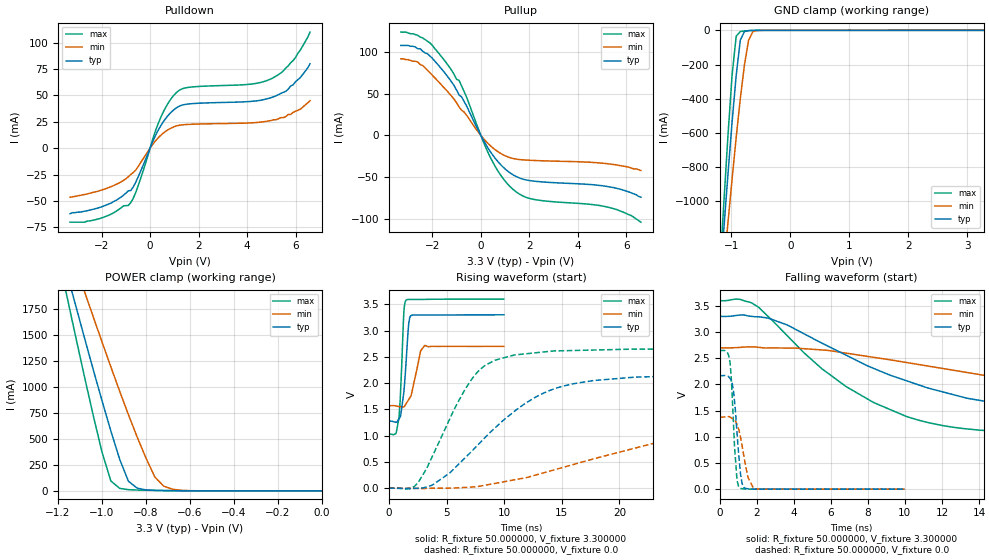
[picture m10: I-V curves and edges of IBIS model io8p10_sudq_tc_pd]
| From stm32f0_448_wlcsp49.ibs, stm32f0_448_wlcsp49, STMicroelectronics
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|   Model io8p10_sudq_tc_pd
[Model]  io8p10_sudq_tc_pd
Model_type I/O
Polarity   Non-Inverting
Enable   Active-Low
Vinl =   0.990000V
Vinh =   2.310000V
Vmeas =  1.650000V
Cref =   50.000000pF
Rref =   100.000000M
Vref =   0.0V
C_comp   1.329900pF   1.255600pF   1.431200pF
[Temperature Range]   25.000000   0.125000k   -40.000000
[Pullup Reference]   3.300000V   2.700000V   3.600000V
[Pulldown Reference]   0.0V   0.0V   0.0V
[POWER Clamp Reference]   3.300000V   2.700000V   3.600000V
[GND Clamp Reference]   0.0V   0.0V   0.0V
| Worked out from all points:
|   slope of the pulldown table from 0 to 0.495 V, typ, clamps not added: 21.3 ohm
|   slope of the pullup table from 0 to 0.495 V, typ, clamps not added: 20.9 ohm
|   GND clamp passes 1 mA (typ) near -0.66 V on its own axis
|   POWER clamp passes 1 mA (typ) near -0.60 V on its own axis
|   rising waveform, R_fixture 50.000000, V_fixture 3.300000: 20-80 % time 430ps typ, 663ps min, 305ps max; typ from 1.27 V to 3.3 V
|   rising waveform, R_fixture 50.000000, V_fixture 0.0: 20-80 % time 6.79ns typ, 16.1ns min, 3.73ns max; typ from 0 V to 2.17 V
|   falling waveform, R_fixture 50.000000, V_fixture 3.300000: 20-80 % time 9.37ns typ, 15.7ns min, 5.83ns max; typ from 3.3 V to 1.27 V
|   falling waveform, R_fixture 50.000000, V_fixture 0.0: 20-80 % time 301ps typ, 442ps min, 235ps max; typ from 2.17 V to 0 V
[Pulldown]
|Voltage   I(typ)   I(min)   I(max)
-3.3V     -62mA      -46.4mA    -70mA
-2.1V     -56.2mA    -40.3mA    -66.8mA
-800mV    -40.04mA   -24.9mA    -51.58mA
-500mV    -27.57mA   -17.6mA    -36.07mA
400mV     19.71mA    11.36mA    27.01mA
700mV     29.83mA    16.93mA    40.97mA
1.1V      38.46mA    21.2mA     53.02mA
1.6V      41.98mA    22.62mA    57.7mA
4.1V      44.26mA    24mA       60.59mA
5V        48mA       26.3mA     65.8mA
5.9V      60mA       34mA       83mA
6.6V      80mA       45mA       110mA
[Pullup]
|Voltage   I(typ)   I(min)   I(max)
-3.3V     108mA      92mA       124mA
-2.6V     104mA      88mA       120mA
-2.2V     98mA       78.2mA     113mA
-1.4V     71.8mA     53.6mA     86.1mA
-900mV    48.51mA    34.23mA    66.14mA
-700mV    41.33mA    28.36mA    53.31mA
400mV     -19.77mA   -12.52mA   -26.8mA
900mV     -37.48mA   -22.89mA   -50.99mA
1.4V      -48.39mA   -28.06mA   -66.43mA
2.2V      -54.79mA   -29.98mA   -76.75mA
5.3V      -61.7mA    -34.2mA    -86.4mA
6.6V      -74mA      -42mA      -104mA
[GND_clamp]
|Voltage   I(typ)   I(min)   I(max)
-3.3V     -9.739A    -9.975A    -9.587A
-1.2V     -1.489A    -1.65A     -1.416A
-1.13V    -1.162A    -1.385A    -1.009A
-1.06V    -842.3mA   -1.125A    -616.9mA
-990mV    -537.1mA   -870.2mA   -263mA
-920mV    -262.5mA   -625.3mA   -33.98mA
-850mV    -56.96mA   -397.5mA   -7.097mA
-780mV    -7.026mA   -202.3mA   -3.727mA
-710mV    -1.792mA   -58.24mA   -1.753mA
-640mV    -564.1uA   -8.795mA   -558.4uA
-570mV    -123.3uA   -1.303mA   -102.2uA
3.28V     84.11uA    64.12uA    93.81uA
[POWER_clamp]
|Voltage   I(typ)   I(min)   I(max)
-3.28V    9.897A     9.838A     9.594A
-1.16V    2.103A     2.419A     1.88A
-1.12V    1.788A     2.17A      1.488A
-1.08V    1.476A     1.923A     1.102A
-1V       868.1mA    1.435A     373.1mA
-960mV    578.2mA    1.196A     96.06mA
-880mV    93.24mA    734.1mA    12.01mA
-840mV    26.3mA     517.4mA    8.56mA
-760mV    5.106mA    134mA      5.119mA
-720mV    3.355mA    46.34mA    3.808mA
-600mV    1.005mA    2.564mA    1.072mA
0V        0A         0A         0A
[Ramp]
| variable   typ   min   max
dV/dt_r  1.29960/6.77882n   0.81036/16.38939n   1.58808/3.72470n
dV/dt_f  1.21482/9.36459n   0.67020/15.73370n   1.54218/5.82341n
R_load = 50.000000
[Rising Waveform]
R_fixture= 50.000000
V_fixture= 3.300000
V_fixture_min= 2.700000
V_fixture_max= 3.600000
|time   V(typ)   V(min)   V(max)
0s        1.274V     1.569V     1.029V
620.6ps   1.256V     1.566V     1.041V
860.9ps   1.315V     1.553V     1.315V
981ps     1.358V     1.549V     1.676V
1.301ns   1.832V     1.546V     3.346V
1.481ns   2.358V     1.603V     3.576V
1.822ns   3.255V     1.723V     3.592V
2.763ns   3.296V     2.617V     3.591V
3.123ns   3.295V     2.718V     3.593V
9.97ns    3.299V     2.699V     3.599V
[Rising Waveform]
R_fixture= 50.000000
V_fixture= 0.0
V_fixture_min= 0.0
V_fixture_max= 0.0
|time   V(typ)   V(min)   V(max)
0s        1.008nV    9.499nV    1.541nV
2.503ns   -533uV     -4.777mV   100.4mV
3.804ns   64.16mV    -612.1uV   621.4mV
7.307ns   729mV      24.19mV    2.109V
8.408ns   978.5mV    59.41mV    2.344V
10.81ns   1.449V     156.4mV    2.531V
14.01ns   1.865V     329.1mV    2.606V
17.82ns   2.05V      562.2mV    2.63V
32.93ns   2.159V     1.214V     2.647V
49.85ns   2.166V     1.377V     2.647V
[Falling Waveform]
R_fixture= 50.000000
V_fixture= 3.300000
V_fixture_min= 2.700000
V_fixture_max= 3.600000
|time   V(typ)   V(min)   V(max)
0s        3.299V     2.699V     3.599V
1.101ns   3.325V     2.708V     3.624V
2.002ns   3.292V     2.713V     3.497V
5.506ns   2.791V     2.659V     2.303V
8.308ns   2.306V     2.518V     1.654V
12.61ns   1.804V     2.271V     1.182V
17.62ns   1.485V     2.026V     1.069V
22.32ns   1.359V     1.854V     1.043V
30.73ns   1.293V     1.679V     1.031V
49.85ns   1.274V     1.569V     1.029V
[Falling Waveform]
R_fixture= 50.000000
V_fixture= 0.0
V_fixture_min= 0.0
V_fixture_max= 0.0
|time   V(typ)   V(min)   V(max)
0s        2.166V     1.377V     2.647V
400.4ps   2.159V     1.383V     2.614V
560.6ps   2.112V     1.375V     2.411V
740.7ps   1.887V     1.333V     1.279V
920.9ps   1.15V      1.242V     236.5mV
1.081ns   455.4mV    1.062V     25.44mV
1.301ns   34.74mV    639.5mV    3.753mV
1.522ns   6.625mV    236.2mV    1.069mV
1.842ns   898.4uV    6.061mV    849.1uV
9.97ns    1.008nV    9.499nV    1.541nV
